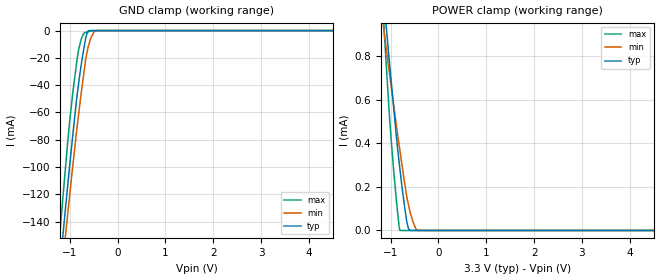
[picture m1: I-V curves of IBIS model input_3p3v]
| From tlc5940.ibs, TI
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|   input_3p3v Model
[Model]   input_3p3v
Model_type   Input
Vinl = 0.66
Vinh = 2.64
C_comp   1.224e-12   1.222e-12   1.241e-12
[Model Spec]
Vinl   0.66   0.6   0.72
Vinh   2.64   2.4   2.88
[Voltage Range]   3.3   3   3.6
|Ambient Temperature   25   85   -40
|Junction Temperature
[Temperature Range]   65   125   -40
[Power Clamp Reference]   3.3   3   3.6
[GND Clamp Reference]   0   0   0
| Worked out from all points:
|   GND clamp passes 1 mA (typ) near -0.63 V on its own axis
|   POWER clamp passes 1 mA (typ) near -1.12 V on its own axis
[GND Clamp]
|   Voltage   I(typ)   I(min)   I(max)
-3.3V     -1.048A    -1A        -1.104A
-1.224V   -180.9mA   -197.7mA   -156.7mA
-1.162V   -157.3mA   -175.9mA   -130.3mA
-1.082V   -128.1mA   -148.3mA   -97.98mA
-1.068V   -122.9mA   -143.3mA   -92.19mA
-934.8mV  -76.5mA    -99mA      -45.41mA
-819.6mV  -40.33mA   -63.01mA   -14.9mA
-722.4mV  -16.93mA   -35.92mA   -3.138mA
-615mV    -166.7uA   -12.19mA   -876.3uA
-495mV    0A         -1.118mA   0A
-414mV    0A         0A         0A
6.6V      0A         0A         0A
[POWER Clamp]
|   Voltage   I(typ)   I(min)   I(max)
-3.3V     6.66mA     4.782mA    9.228mA
-1.162V   1.111mA    958uA      1.015mA
-1.126V   1.022mA    896.2uA    885.7uA
-1.059V   857.4uA    781.8uA    649.7uA
-1.018V   757.8uA    712.1uA    504.9uA
-931.2mV  553.7uA    568.6uA    264uA
-808.8mV  289.3uA    372.3uA    1.111uA
-706.2mV  107.7uA    218.2uA    0A
-623.7mV  7.79uA     114.9uA    0A
-534mV    0A         41.41uA    0A
-420mV    0A         0A         0A
6.6V      0A         0A         0A
